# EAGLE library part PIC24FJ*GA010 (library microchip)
64/80/100-Pin General Purpose, 16-Bit Flash Microcontrollers Source: http://ww1.microchip.com/downloads/en/DeviceDoc/39747d.pdf
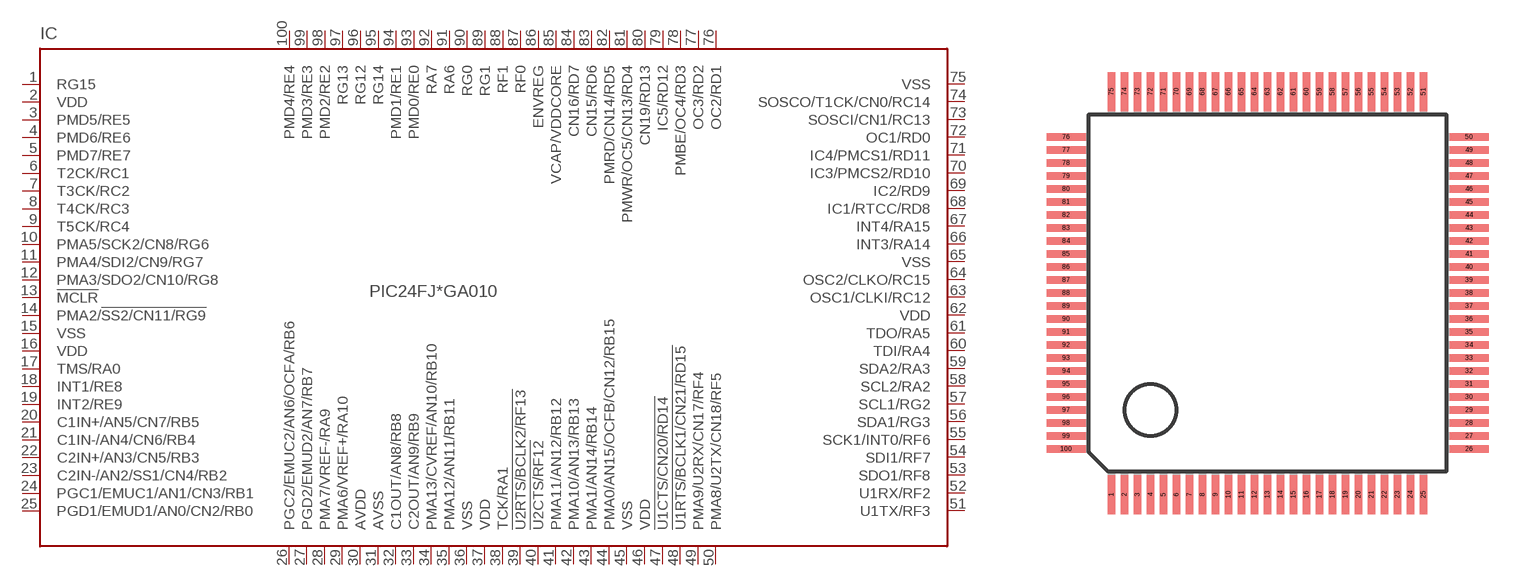
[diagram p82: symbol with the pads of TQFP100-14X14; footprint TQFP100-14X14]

Designator prefix IC

## PIC24FJ128GA010 (MPN: PIC24FJ128GA010-I/PT; OC_FARNELL: 1146522; OC_NEWARK: 56K7341), PIC24FJ64GA010 (MPN: PIC24FJ64GA010-I/PT; OC_FARNELL: 1146526; OC_NEWARK: 56K7347), PIC24FJ96GA010 (MPN: PIC24FJ96GA010-I/PT; OC_FARNELL: 1778488; OC_NEWARK: 56K7353)  [TQFP100-14X14]
1  RG15
2  VDD  pwr
3  PMD5/RE5
4  PMD6/RE6
5  PMD7/RE7
6  T2CK/RC1
7  T3CK/RC2
8  T4CK/RC3
9  T5CK/RC4
10  PMA5/SCK2/CN8/RG6
11  PMA4/SDI2/CN9/RG7
12  PMA3/SDO2/CN10/RG8
13  !MCLR
14  PMA2/!SS2/CN11/RG9
15  VSS  pwr
16  VDD  pwr
17  TMS/RA0
18  INT1/RE8
19  INT2/RE9
20  C1IN+/AN5/CN7/RB5
21  C1IN-/AN4/CN6/RB4
22  C2IN+/AN3/CN5/RB3
23  C2IN-/AN2/SS1/CN4/RB2
24  PGC1/EMUC1/AN1/CN3/RB1
25  PGD1/EMUD1/AN0/CN2/RB0
26  PGC2/EMUC2/AN6/OCFA/RB6
27  PGD2/EMUD2/AN7/RB7
28  PMA7/VREF-/RA9
29  PMA6/VREF+/RA10
30  AVDD  pwr
31  AVSS  pwr
32  C1OUT/AN8/RB8
33  C2OUT/AN9/RB9
34  PMA13/CVREF/AN10/RB10
35  PMA12/AN11/RB11
36  VSS  pwr
37  VDD  pwr
38  TCK/RA1
39  !U2RTS/BCLK2/RF13
40  !U2CTS/RF12
41  PMA11/AN12/RB12
42  PMA10/AN13/RB13
43  PMA1/AN14/RB14
44  PMA0/AN15/OCFB/CN12/RB15
45  VSS  pwr
46  VDD  pwr
47  !U1CTS/CN20/RD14
48  !U1RTS/BCLK1/CN21/RD15
49  PMA9/U2RX/CN17/RF4
50  PMA8/U2TX/CN18/RF5
51  U1TX/RF3
52  U1RX/RF2
53  SDO1/RF8
54  SDI1/RF7
55  SCK1/INT0/RF6
56  SDA1/RG3
57  SCL1/RG2
58  SCL2/RA2
59  SDA2/RA3
60  TDI/RA4
61  TDO/RA5
62  VDD  pwr
63  OSC1/CLKI/RC12
64  OSC2/CLKO/RC15
65  VSS  pwr
66  INT3/RA14
67  INT4/RA15
68  IC1/RTCC/RD8
69  IC2/RD9
70  IC3/PMCS2/RD10
71  IC4/PMCS1/RD11
72  OC1/RD0
73  SOSCI/CN1/RC13
74  SOSCO/T1CK/CN0/RC14
75  VSS  pwr
76  OC2/RD1
77  OC3/RD2
78  PMBE/OC4/RD3
79  IC5/RD12
80  CN19/RD13
81  PMWR/OC5/CN13/RD4
82  PMRD/CN14/RD5
83  CN15/RD6
84  CN16/RD7
85  VCAP/VDDCORE
86  ENVREG
87  RF0
88  RF1
89  RG1
90  RG0
91  RA6
92  RA7
93  PMD0/RE0
94  PMD1/RE1
95  RG14
96  RG12
97  RG13
98  PMD2/RE2
99  PMD3/RE3
100  PMD4/RE4

## Footprint TQFP100-14X14 (pad centres in mm)
Thin Quad Flat Pack 14x14 mm
smd 0.27 x 1.5: 1 -6,-7.75; 2 -5.5,-7.75; 3 -5,-7.75; 4 -4.5,-7.75; 5 -4,-7.75; 6 -3.5,-7.75; 7 -3,-7.75; 8 -2.5,-7.75; 9 -2,-7.75; 10 -1.5,-7.75; 11 -1,-7.75; 12 -0.5,-7.75; 13 0,-7.75; 14 0.5,-7.75; 15 1,-7.75; 16 1.5,-7.75; 17 2,-7.75; 18 2.5,-7.75; 19 3,-7.75; 20 3.5,-7.75; 21 4,-7.75; 22 4.5,-7.75; 23 5,-7.75; 24 5.5,-7.75; 25 6,-7.75; 51 6,7.75; 52 5.5,7.75; 53 5,7.75; 54 4.5,7.75; 55 4,7.75; 56 3.5,7.75; 57 3,7.75; 58 2.5,7.75; 59 2,7.75; 60 1.5,7.75; 61 1,7.75; 62 0.5,7.75; 63 0,7.75; 64 -0.5,7.75; 65 -1,7.75; 66 -1.5,7.75; 67 -2,7.75; 68 -2.5,7.75; 69 -3,7.75; 70 -3.5,7.75; 71 -4,7.75; 72 -4.5,7.75; 73 -5,7.75; 74 -5.5,7.75; 75 -6,7.75
smd 1.5 x 0.27: 26 7.75,-6; 27 7.75,-5.5; 28 7.75,-5; 29 7.75,-4.5; 30 7.75,-4; 31 7.75,-3.5; 32 7.75,-3; 33 7.75,-2.5; 34 7.75,-2; 35 7.75,-1.5; 36 7.75,-1; 37 7.75,-0.5; 38 7.75,0; 39 7.75,0.5; 40 7.75,1; 41 7.75,1.5; 42 7.75,2; 43 7.75,2.5; 44 7.75,3; 45 7.75,3.5; 46 7.75,4; 47 7.75,4.5; 48 7.75,5; 49 7.75,5.5; 50 7.75,6; 76 -7.75,6; 77 -7.75,5.5; 78 -7.75,5; 79 -7.75,4.5; 80 -7.75,4; 81 -7.75,3.5; 82 -7.75,3; 83 -7.75,2.5; 84 -7.75,2; 85 -7.75,1.5; 86 -7.75,1; 87 -7.75,0.5; 88 -7.75,0; 89 -7.75,-0.5; 90 -7.75,-1; 91 -7.75,-1.5; 92 -7.75,-2; 93 -7.75,-2.5; 94 -7.75,-3; 95 -7.75,-3.5; 96 -7.75,-4; 97 -7.75,-4.5; 98 -7.75,-5; 99 -7.75,-5.5; 100 -7.75,-6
